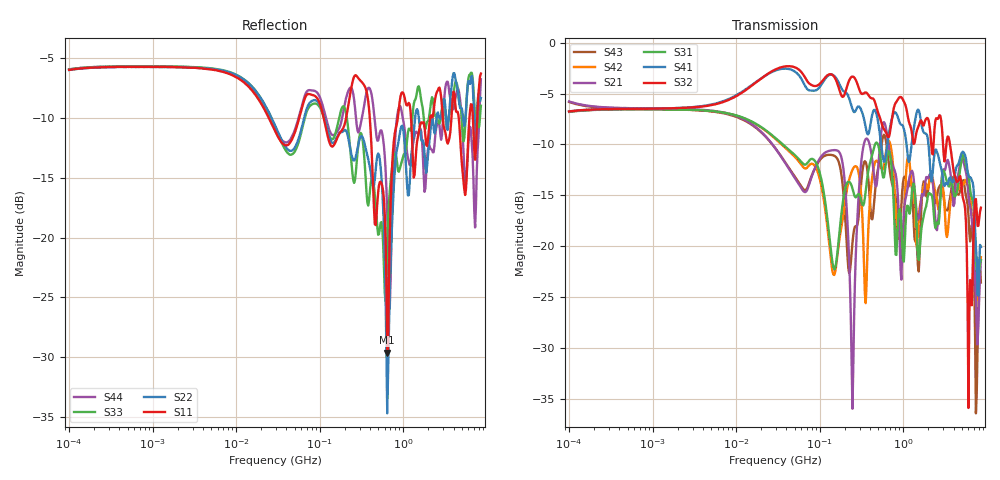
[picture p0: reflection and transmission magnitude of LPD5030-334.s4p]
# MHz S MA R 50
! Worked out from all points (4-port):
!   498 points, 100 kHz to 8.5 GHz, reference 50 ohm
!   strongest paths, dB at 100 kHz, 1.698 MHz, 29.49 MHz, 500.7 MHz, 8.5 GHz:
!     S32: -6.8, -6.4, -2.6, -6.9, -16.2
!     S41: -6.8, -6.4, -2.7, -7.8, -20.1
!     S31: -6.8, -6.5, -9.4, -10.1, -21.4
!     S21: -5.8, -6.5, -10.4, -12.4, -21.4
!     S42: -6.8, -6.6, -9.4, -11.7, -21.1
!     S43: -5.8, -6.6, -10.4, -12.4, -23.6
!   lowest |S11| = -29.6 dB at 643.6 MHz (marker M1), VSWR 1.07, Z = 48.8 - j3.04 ohm
!   |S11| at or under -10 dB: 1.239 GHz to 2.099 GHz (860.2 MHz wide, 51.6 % of centre); 2.977 GHz to 3.772 GHz (795.6 MHz wide, 23.6 % of centre); 4.616 GHz to 6.199 GHz (1.583 GHz wide, 29.3 % of centre)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
0.1  0.5035 12.1  0.515 -12.5  0.4578 -166.8  0.4596 13.8
     0.515 -12.5  0.5021 12.1  0.4594 13.8  0.4578 -166.9
     0.4578 -166.8  0.4594 13.8  0.5054 12.1  0.5114 -12.5
     0.4596 13.8  0.4578 -166.9  0.5114 -12.5  0.505 12.2
167.2873  0.2673 -17.9  0.2931 16.5  0.1035 136.4  0.6417 -44.3
          0.2931 16.5  0.2707 -34.8  0.6088 -38.8  0.09873 127.4
          0.1035 136.4  0.6088 -38.8  0.3065 -28.1  0.2624 18.1
          0.6417 -44.3  0.09873 127.4  0.2624 18.1  0.2829 -18.1
246.6465  0.4471 -27.7  0.01588 8.7  0.1922 21.5  0.4722 -59.3
          0.01588 8.7  0.2145 -53.8  0.6821 -44.7  0.2375 29.9
          0.1922 21.5  0.6821 -44.7  0.1853 -65.4  0.1038 26.4
          0.4722 -59.3  0.2375 29.9  0.1038 26.4  0.413 -44.8
331.9048  0.4399 -72.3  0.3065 25.9  0.1585 4.9  0.4371 -71.9
          0.3065 25.9  0.2587 -67.9  0.562 -61.9  0.1092 -46.3
          0.1585 4.9  0.562 -61.9  0.2431 -78.8  0.2489 8.8
          0.4371 -71.9  0.1092 -46.3  0.2489 8.8  0.339 -42.9
643.6438  0.03296 -109.6  0.3485 -89.9  0.2836 -82.2  0.3158 -83.2
          0.3485 -89.9  0.01836 86.9  0.3501 -98.5  0.3163 -66.6
          0.2836 -82.2  0.3501 -98.5  0.09429 -32.6  0.2961 -89.2
          0.3158 -83.2  0.3163 -66.6  0.2961 -89.2  0.1246 -140.3
948.981  0.4015 -110.9  0.06852 -116.6  0.1287 -140.7  0.3954 -143.3
         0.06852 -116.6  0.292 -101.7  0.5393 -140.8  0.1032 -118.5
         0.1287 -140.7  0.5393 -140.8  0.205 -99.7  0.1574 -97.4
         0.3954 -143.3  0.1032 -118.5  0.1574 -97.4  0.3417 -131.2
8500  0.4854 -52.5  0.08521 34.3  0.08536 -8.3  0.09907 -33.7
      0.08521 34.3  0.3836 -33.8  0.1547 -15.9  0.08829 -6.4
      0.08536 -8.3  0.1547 -15.9  0.3559 -0.8  0.06627 20.1
      0.09907 -33.7  0.08829 -6.4  0.06627 20.1  0.4597 -28.2
